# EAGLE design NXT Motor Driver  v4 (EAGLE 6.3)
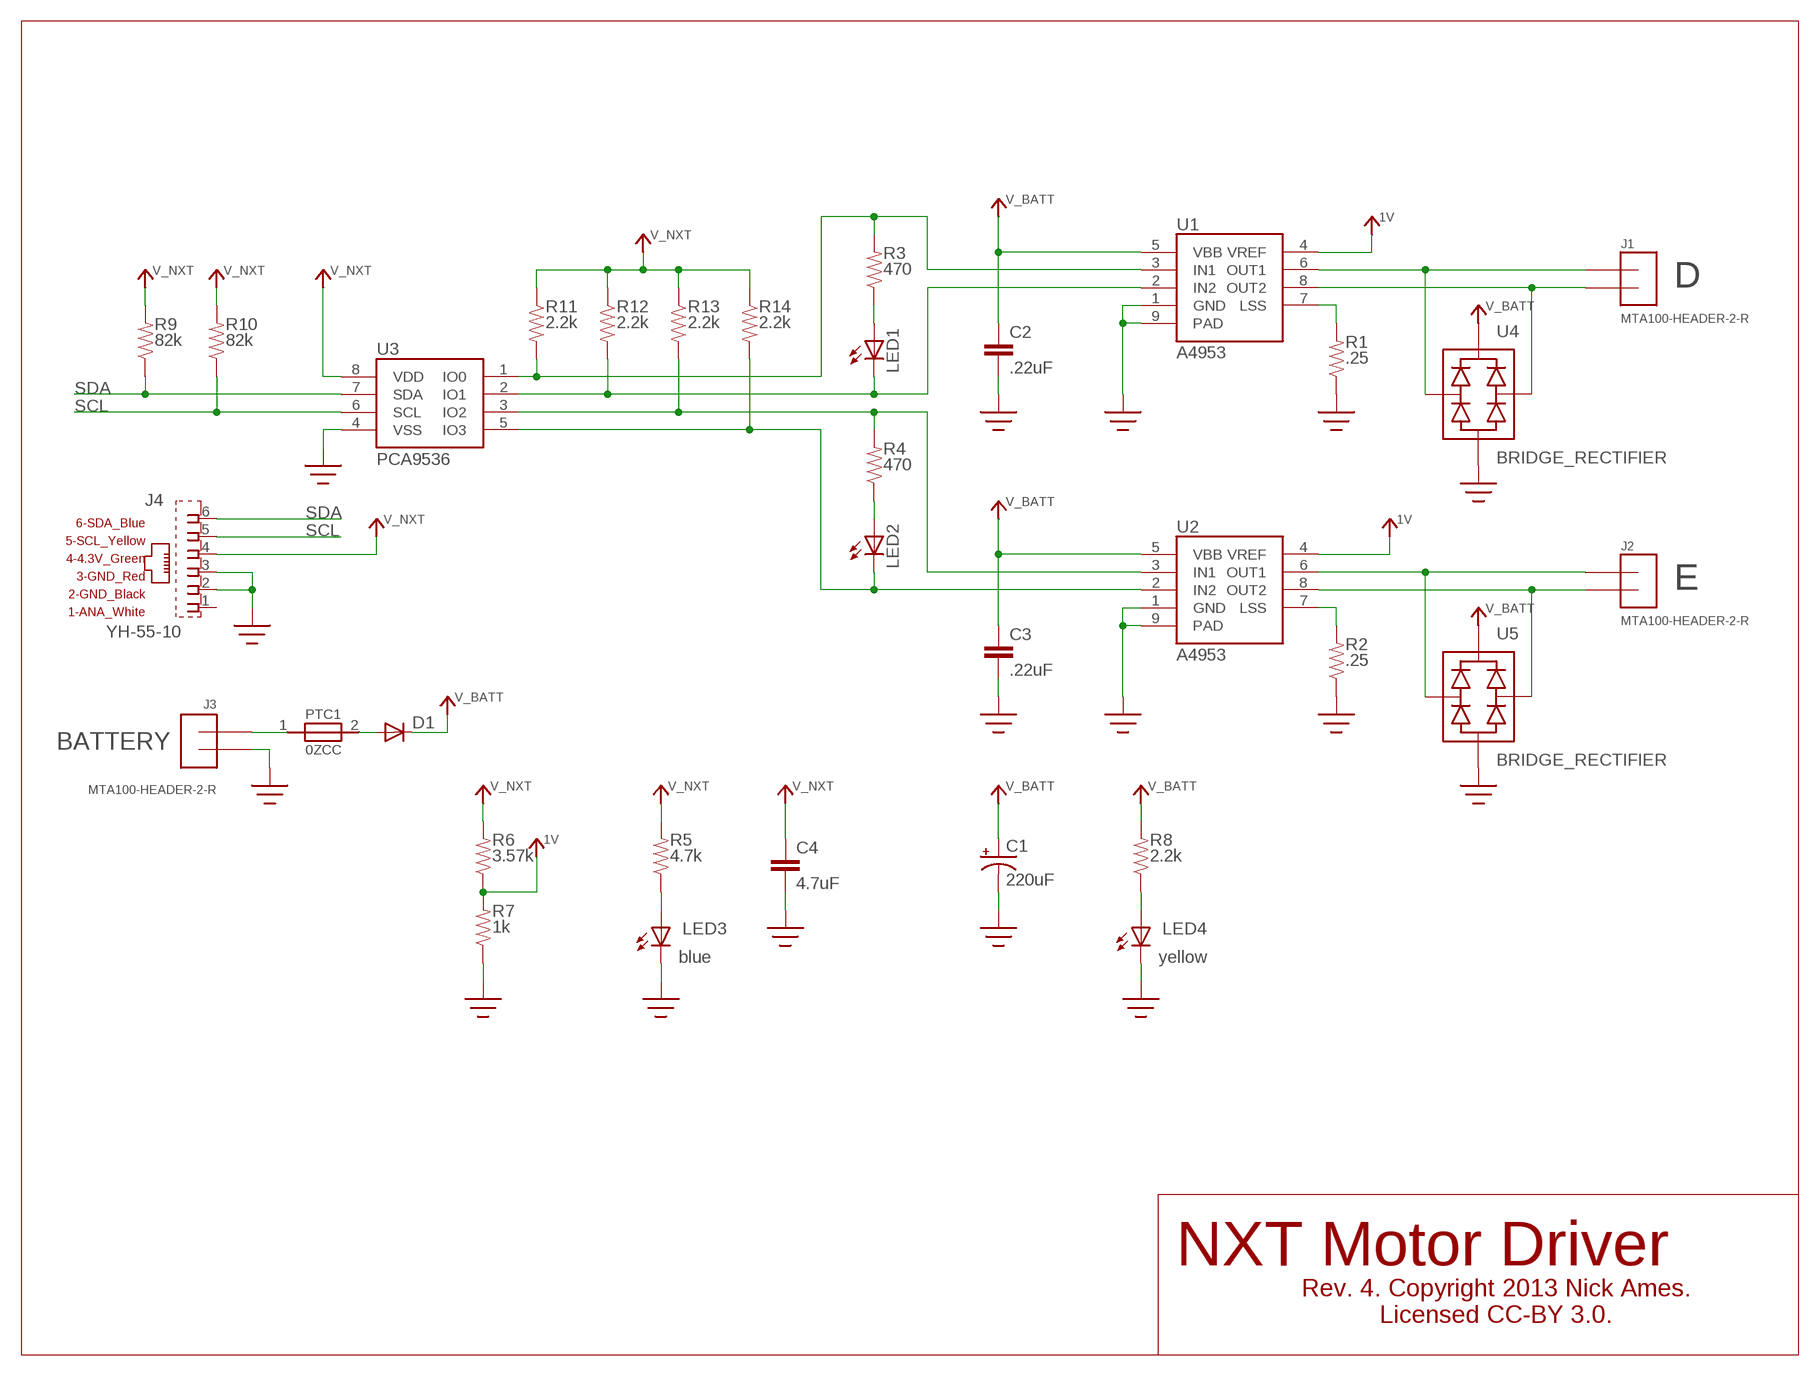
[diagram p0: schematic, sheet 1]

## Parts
C1  220uF  CAP_POL  [CAPACITOR-197]
C2  .22uF  CAP0603-CAP  [0603-CAP]
C3  .22uF  CAP0603-CAP  [0603-CAP]
C4  4.7uF  CAP0603-CAP  [0603-CAP]
D1  DIODESOD-123LF  [SOD-123LF]
J1  MTA100-HEADER-2-R  [MTA100-HEADER-2-R]
J2  MTA100-HEADER-2-R  [MTA100-HEADER-2-R]
J3  MTA100-HEADER-2-R  [MTA100-HEADER-2-R]
J4  YH-55-10  [YH-55-10]
LED1  LED5MM  [LED5MM]
LED2  LED5MM  [LED5MM]
LED3  LED5MM  [LED5MM]
LED4  LED5MM  [LED5MM]
PTC1  0ZCC  [0ZCC]
R1  .25  RESISTOR  [RESISTOR-2010]
R2  .25  RESISTOR  [RESISTOR-2010]
R3  470  RESISTOR0603-RES  [0603-RES]
R4  470  RESISTOR0603-RES  [0603-RES]
R5  4.7k  RESISTOR0603-RES  [0603-RES]
R6  3.57k  RESISTOR0603-RES  [0603-RES]
R7  1k  RESISTOR0603-RES  [0603-RES]
R8  2.2k  RESISTOR0603-RES  [0603-RES]
R9  82k  RESISTOR0603-RES  [0603-RES]
R10  82k  RESISTOR0603-RES  [0603-RES]
R11  2.2k  RESISTOR0603-RES  [0603-RES]
R12  2.2k  RESISTOR0603-RES  [0603-RES]
R13  2.2k  RESISTOR0603-RES  [0603-RES]
R14  2.2k  RESISTOR0603-RES  [0603-RES]
U1  A4953  [SOIC8-150-PAD-ALLEGRO]
U2  A4953  [SOIC8-150-PAD-ALLEGRO]
U3  PCA9536  [SOIC8-150-JEDEC/IPC]
U4  BRIDGE_RECTIFIER  [SOIC4]
U5  BRIDGE_RECTIFIER  [SOIC4]

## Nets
1V: R6.1 R7.2 U1.4(VREF) U2.4(VREF)
GND: C1.2(-) C2.2 C3.2 C4.2 J3.2 J4.2(2_GND_BLACK) J4.3(3_GND_RED) LED3.K(C) LED4.K(C) R1.P$1 R2.P$1 R7.1 U1.1(GND) U1.9(PAD) U2.1(GND) U2.9(PAD) U3.4(VSS) U4.- U5.-
N$1: R2.P$2 U2.7(LSS)
N$2: R1.P$2 U1.7(LSS)
N$3: J1.1 U1.8(OUT2) U4.AC2
N$4: J1.2 U1.6(OUT1) U4.AC1
N$5: J2.2 U2.6(OUT1) U5.AC1
N$6: J2.1 U2.8(OUT2) U5.AC2
N$7: LED1.A R3.1
N$8: LED2.A R4.1
N$9: R4.2 R13.2 U2.3(IN1) U3.3(IO2)
N$10: R3.2 R11.2 U1.3(IN1) U3.1(IO0)
N$11: LED2.K(C) R14.2 U2.2(IN2) U3.5(IO3)
N$12: LED4.A R8.1
N$13: LED3.A R5.1
N$14: LED1.K(C) R12.2 U1.2(IN2) U3.2(IO1)
N$15: J3.1 PTC1.1
N$16: D1.+(A) PTC1.2
SCL: J4.5(5_SCL_YELLOW) R10.1 U3.6(SCL)
SDA: J4.6(6_SDA_BLUE) R9.1 U3.7(SDA)
V_BATT: C1.1(+) C2.1 C3.1 D1.-(C) R8.2 U1.5(VBB) U2.5(VBB) U4.+ U5.+
V_NXT: C4.1 J4.4(4_4.3V_GREEN) R5.2 R6.2 R9.2 R10.2 R11.1 R12.1 R13.1 R14.1 U3.8(VDD)
Unconnected: J4.1(1_ANA_WHITE)

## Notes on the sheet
- D
- E
- BATTERY
- blue | yellow
- NXT Motor Driver
- Rev. 4. Copyright 2013 Nick Ames.
  Licensed CC-BY 3.0.

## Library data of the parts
C1 = NA-lib:CAP_POL: Capacitor Polarized
C2-C4 = SparkFun:CAP: Capacitor
D1 = NA-lib:DIODE: Diode
J1-J3 = NA-lib:MTA100-HEADER-2-R
J4 = Dexter_Industries_Eagle_Library_Female_Sockets:YH-55-10: RJ11 6 connects Source:Dexter Industries LEGO MINDSTORMS NXT Female Adapter; OC_FARNELL: unknown; OC_NEWARK: unknown
LED1-LED4 = SparkFun:LED: LEDs
PTC1 = NA-lib:0ZCC
R1-R4 R9 R10 = NA-lib:RESISTOR: Resistor
R5-R8 R11-R14 = SparkFun:RESISTOR: Resistor
U1 U2 = NA-lib:A4953
U3 = NA-lib:PCA9536
U4 U5 = NA-lib:BRIDGE_RECTIFIER

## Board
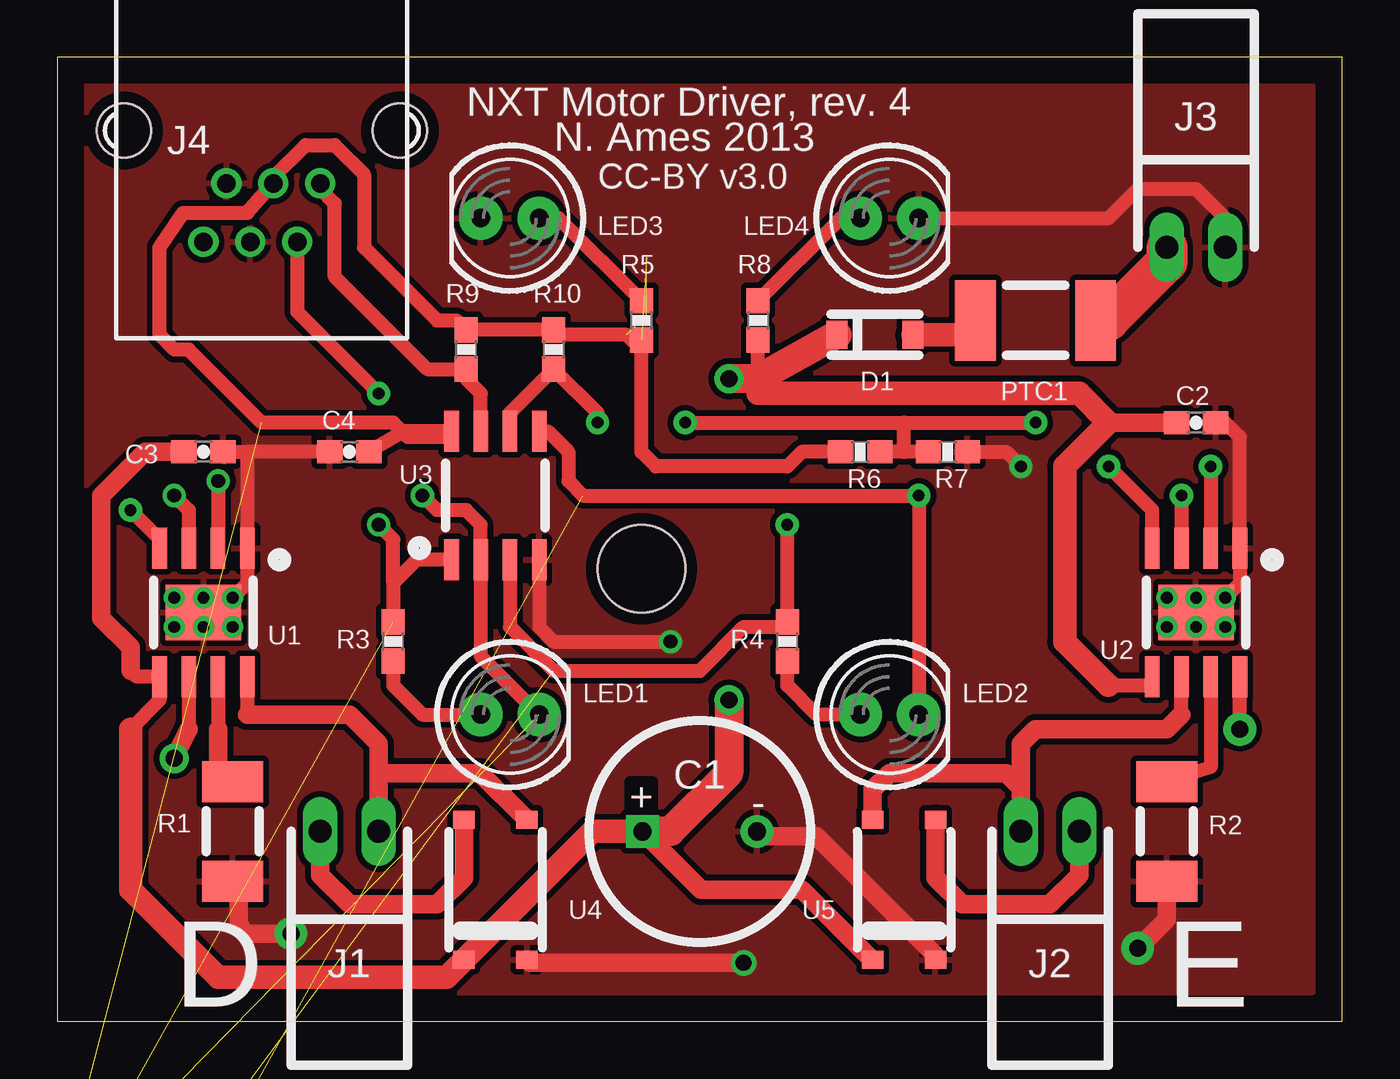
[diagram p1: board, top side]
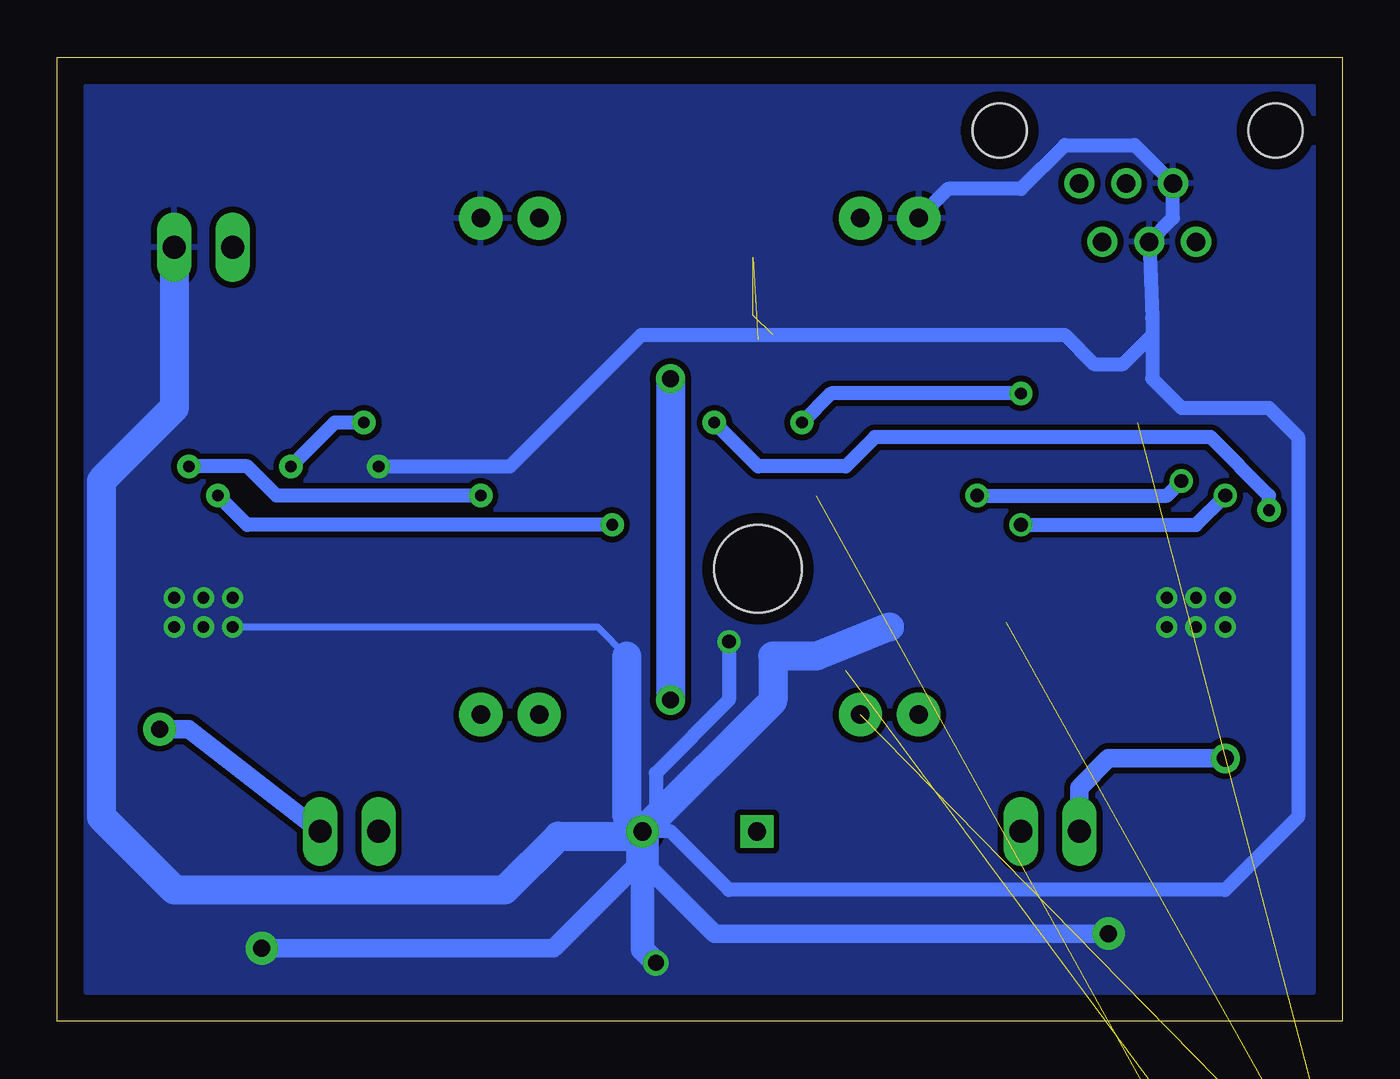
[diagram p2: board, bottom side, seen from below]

Size 55.88 x 41.91 mm. Coordinates in mm from the lower left corner, seen from the top.
Outline: 0,0 55.88,0 55.88,41.91 0,41.91 0,0
Copper layers (1*16): Top 0.035mm / dielectric 1.5mm / Bottom 0.035mm
Design rules "default *": minimum track width 9mil, minimum drill 13mil, track to track 10mil, track to pad 10mil, pad to pad 10mil, via to via 10mil, smd to smd 0mil, copper to edge 20mil, drill to drill 20mil, minimum pad ring 10mil, minimum via ring 8mil, stop-mask expansion 4mil, vias tented up to drill 30mil, thermal gap 10mil
Holes 3.81 mm at 25.4,19.68

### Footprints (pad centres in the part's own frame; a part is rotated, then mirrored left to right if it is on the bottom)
CAPACITOR-197 = drill 0.8 pad 1.422 square: 1 -2.489,0 | drill 0.8 pad 1.422: 2 2.489,0
0603-CAP = smd 1.1 x 1: 1 -0.85,0; 2 0.85,0
SOD-123LF = smd 0.914 x 1.219: + 1.651,0; - -1.651,0
MTA100-HEADER-2-R = drill 1 pad 1.422 long: 1 0,1.27; 2 0,-1.27
YH-55-10 = drill 0.8 pad 1.3: 1 2.54,4.84; 2 1.54,2.3; 3 0.5,4.84; 4 -0.5,2.3; 5 -1.54,4.84; 6 -2.54,2.3 | hole 2.36: -6,0; 6,0
LED5MM = drill 0.813 pad 1.88: A -1.27,0; K 1.27,0
0ZCC = smd 1.778 x 3.505: 1 -2.616,0; 2 2.616,0
RESISTOR-2010 = smd 1.778 x 2.667: P$1 -2.159,0; P$2 2.159,0
0603-RES = smd 1.1 x 1: 1 -0.85,0; 2 0.85,0
SOIC8-150-PAD-ALLEGRO = smd 0.635 x 1.778: 1 -1.905,-2.794; 2 -0.635,-2.794; 3 0.635,-2.794; 4 1.905,-2.794; 5 1.905,2.794; 6 0.635,2.794; 7 -0.635,2.794; 8 -1.905,2.794 | smd 3.302 x 2.413: 9 0,0
SOIC8-150-JEDEC/IPC = smd 0.635 x 1.778: 1 -1.905,-2.794; 2 -0.635,-2.794; 3 0.635,-2.794; 4 1.905,-2.794; 5 1.905,2.794; 6 0.635,2.794; 7 -0.635,2.794; 8 -1.905,2.794
SOIC4 = smd 0.94 x 0.787: + -1.372,-3.048; - 1.372,-3.048; AC1 -1.372,3.048; AC2 1.372,3.048

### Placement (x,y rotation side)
C1  27.94,8.26 0 top
C2  49.53,26.04 0 top
C3  6.35,24.77 0 top
C4  12.7,24.77 180 top
D1  35.56,29.84 0 top
J1  12.7,8.26 270 top
J2  43.18,8.26 270 top
J3  49.53,33.66 90 top
J4  8.89,38.73 180 top
LED1  19.68,13.34 0 top
LED2  36.2,13.34 0 top
LED3  19.68,34.92 180 top
LED4  36.2,34.92 0 top
PTC1  42.55,30.48 180 top
R1  7.62,8.26 90 top
R2  48.26,8.26 90 top
R3  14.61,16.51 90 top
R4  31.75,16.51 90 top
R5  25.4,30.48 270 top
R6  34.92,24.77 180 top
R7  38.73,24.77 180 top
R8  30.48,30.48 270 top
R9  17.78,29.21 90 top
R10  21.59,29.21 90 top
R11  not placed on the board
R12  not placed on the board
R13  not placed on the board
R14  not placed on the board
U1  6.35,17.78 180 top
U2  49.53,17.78 180 top
U3  19.05,22.86 0 top
U4  19.05,5.71 0 top
U5  36.83,5.71 0 top

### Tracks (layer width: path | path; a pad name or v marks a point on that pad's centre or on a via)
1V  (via drill 0.51 pad 1.02)
  Top 0.61: U2.4 47.62,22.23 v45.72,24.13 | 36.83,24.77 R6.1 | R7.2 36.83,24.77 | U1.4 4.45,20.95 v3.17,22.23 | v27.3,26.04 36.83,26.04 | 36.83,24.77 36.83,26.04 | 36.83,26.04 v42.55,26.04
  Bottom 0.61: v3.17,22.23 3.17,22.86 5.71,25.4 20.32,25.4 21.59,24.13 25.4,24.13 v27.3,26.04 | v42.55,26.04 43.81,26.04 v45.72,24.13
GND  (via drill 0.51, 0.51 pad 0.25, 0.51 pad 1.02, 0.6, 0.7, 0.74 pad 1.42)
  Top 0.254: U1.9 6.99,17.78 6.99,17.14
  Top 0.305: U2.9 48.9,17.78 v48.26,17.14
  Top 0.61: U3.4 20.95,17.14 21.59,16.51 v26.67,16.51 | C4.2 8.26,24.77 | 8.26,24.77 U1.1 8.26,19.05 v7.62,18.41 6.99,17.78 | C2.2 50.8,26.04 51.44,25.4 U2.1 51.44,19.05 v50.8,18.41 50.16,18.41 U2.9 | C3.2 8.26,24.77 | R7.1 41.27,24.77 v41.91,24.13 | J3.2 50.8,34.92 49.53,36.2 46.99,36.2 45.72,34.92 LED4.K
  Top 0.813: U5.- 38.2,2.87 33.02,8.05 30.63,8.05 C1.2 | v29.84,2.54 20.55,2.54 U4.- | v46.99,3.17 48.26,4.45 R2.P$1 | 7.87,6.1 7.87,4.19 8.26,3.81 v10.16,3.81
  Top 1.016: R1.P$1 7.87,6.1
  Bottom 0.305: v48.26,17.14 32.38,17.14 31.11,15.88
  Bottom 0.61: v26.67,16.51 26.67,13.97 29.84,10.79 29.84,8.84 C1.2 29.21,8.26 26.67,5.71 5.08,5.71 1.91,8.89 1.91,25.4 3.17,26.67 6.99,26.67 8.26,27.94 8.26,29.84 | 8.26,29.84 8.26,30.59 J4.3 7.35,34.94 J4.2 9.02,38.1 12.06,38.1 13.97,36.2 17.14,36.2 LED3.K | v41.91,24.13 36.2,24.13 30.48,29.84 12.06,29.84 10.79,28.57 9.53,28.57 8.26,29.84
  Bottom 0.813: 30.43,6.93 27.3,3.81 v10.16,3.81 | 30.43,7.04 34.29,3.17 v46.99,3.17
  Bottom 1.016: v29.84,2.54 30.43,3.12 30.43,7.62
  Bottom 1.27: 19.68,17.14 22.86,15.88 24.77,15.88 24.77,13.92 C1.2 | 31.11,15.88 31.11,8.94 C1.2 | J3.2 50.8,26.67 53.98,23.5 53.98,8.89 50.8,5.71 36.42,5.71 34.09,8.05 30.63,8.05 C1.2
  Bottom 1.422: 30.43,6.93 30.43,7.04 30.43,7.62 C1.2
  other vias: 5.08,18.41 6.35,18.41 5.08,17.14 6.35,17.14 7.62,17.14 50.8,17.14 49.53,17.14 48.26,18.41 49.53,18.41
  pour Bottom: 3.17,15.24 3.17,20.32 25.27,20.32 25.27,15.24
  pour Bottom: 30.61,15.24 30.61,20.32 52.7,20.32 52.7,15.24
  pour Bottom (isolate 0.254): 54.61,1.27 54.61,40.64 1.27,40.64 1.27,38.1 1.27,1.27
  pour Top (isolate 0.254): 1.27,1.27 54.61,1.27 54.61,40.64 1.27,40.64
N$1
  Top 0.61: U2.7 50.16,11.05 R2.P$2
N$2
  Top 0.61: 6.99,11.05 R1.P$2 | U1.7 6.99,12.7
  Top 0.813: 6.99,12.7 6.99,11.05
N$3
  Top 0.61: U1.8 8.26,13.34
  Top 0.813: 8.26,13.34 12.7,13.34 13.97,12.06 13.97,10.79 | 13.97,10.79 J1.1 | U4.AC2 18.39,10.79 13.97,10.79
N$4  (via drill 0.74 pad 1.27)
  Top 0.61: U1.6 5.71,12.7
  Top 0.813: 5.71,12.7 v5.08,11.43 | U4.AC1 17.68,6.25 16.51,5.08 12.7,5.08 11.43,6.35 J1.2
  Bottom 0.813: v5.08,11.43 10.16,11.43 11.43,10.16 J1.2
N$5
  Top 0.61: 48.9,13.34 U2.6
  Top 0.813: 48.9,13.34 48.26,12.7 42.55,12.7 41.91,12.06 41.91,10.16 | 41.91,10.16 J2.2 | U5.AC1 35.46,10.06 36.2,10.79 41.27,10.79 41.91,10.16
N$6  (via drill 0.74 pad 1.42)
  Top 0.61: v51.44,12.7 U2.8
  Top 0.813: U5.AC2 38.2,6.25 39.37,5.08 43.18,5.08 44.45,6.35 J2.1
  Bottom 0.813: v51.44,12.7 50.16,12.7 J2.1
N$7
  Top 0.61: R3.1 14.61,14.61 15.88,13.34 LED1.A
N$8
  Top 0.61: LED2.A 33.02,13.34 31.75,14.61 R4.1
N$9  (via drill 0.51 pad 1.02)  (1 unrouted)
  Top 0.61: U3.3 19.68,17.14 21.59,15.24 27.94,15.24 29.84,17.14 31.54,17.14 R4.2 v31.75,21.59 | v48.9,22.86 U2.3
  Bottom 0.61: v31.75,21.59 47.62,21.59 v48.9,22.86
N$10  (via drill 0.6)  (1 unrouted)
  Top 0.61: U3.1 15.62,20.07 14.61,19.05 | 14.61,19.05 R3.2 | 14.61,19.05 14.61,20.95 v13.97,21.59 | v5.08,22.86 5.71,22.23 U1.3
  Bottom 0.61: v13.97,21.59 6.35,21.59 v5.08,22.86
N$11  (via drill 0.51 pad 1.02)  (1 unrouted)
  Top 0.61: U3.5 21.34,25.65 22.23,24.77 22.23,23.5 22.86,22.86 v37.47,22.86 LED2.K | v50.16,24.13 U2.2
  Bottom 0.61: v50.16,24.13 47.62,24.13 46.35,22.86 v37.47,22.86
N$12
  Top 0.61: R8.1 34.08,34.92 LED4.A
N$13
  Top 0.61: LED3.A 21.8,34.92 R5.1
N$14  (via drill 0.6)  (1 unrouted)
  Top 0.61: LED1.K 18.41,15.88 U3.2 18.41,21.59 17.78,22.23 16.51,22.23 v15.88,22.86 | v6.99,23.5 U1.2
  Bottom 0.61: v15.88,22.86 7.62,22.86 v6.99,23.5
N$15
  Top 1.778: J3.1 48.26,33.02 45.72,30.48 PTC1.1
N$16
  Top 1.016: PTC1.2 40.01,30.48 40.01,29.84 D1.+
SCL  (via drill 0.51 pad 1.02)
  Top 0.61: v23.5,26.04 23.5,26.45 R10.1 19.68,26.45 U3.6 | J4.5 10.43,30.84 v13.97,27.3
  Bottom 0.61: v13.97,27.3 22.23,27.3 v23.5,26.04
SDA
  Top 0.406: 17.78,27.94 R9.1
  Top 0.61: U3.7 18.41,27.3 17.78,27.94 | R9.1 16.09,28.36 12.06,32.38 12.06,35.56 11.43,36.2 J4.6
V_BATT  (via drill 0.74 pad 1.27)
  Top 0.61: 3.17,12.7 4.45,13.97 U1.5 3.43,14.99 3.17,15.24 | 30.48,27.94 R8.2 | 30.48,27.3 29.84,27.94 | 45.72,14.61 47.62,14.61 U2.5
  Top 0.813: C3.1 3.81,24.77 1.91,22.86 1.91,17.53 3.17,16.26 3.17,15.24 | C2.1 45.72,26.04 | U5.+ 35.43,2.67 32.38,5.71 27.99,5.71 C1.1
  Top 1.016: 25.45,8.2 C1.1 23.27,8.26 U4.+ 16.92,1.91 6.99,1.91 3.17,5.71 3.17,12.7 | 30.48,27.3 44.45,27.3 45.72,26.04 43.81,24.13 43.81,16.51 45.72,14.61
  Top 1.27: D1.- 30.48,27.94 29.84,27.94 v29.21,27.94 | v29.21,13.97 29.21,10.79 26.67,8.26 C1.1
  Bottom 1.27: v29.21,27.94 v29.21,13.97
V_NXT  (7 unrouted)
  Top 0.61: C4.1 15.07,25.65 U3.8 16.89,25.4 15.24,25.4 14.61,26.04 8.89,26.04 5.71,29.21 5.08,29.21 4.45,29.84 4.45,33.66 5.46,35.15 8.26,35.15 J4.4 9.39,36.7 10.79,38.1 12.06,38.1 13.34,36.83 13.34,33.66 16.51,30.48 17.36,30.48 R9.2 R10.2 21.8,29.84 24.77,29.84 25.4,29.21 25.4,24.77 26.04,24.13 31.75,24.13 32.38,24.77 R6.2

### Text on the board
tPlace: NXT Motor Driver, rev. 4 | N. Ames 2013 | CC-BY v3.0 | D | E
